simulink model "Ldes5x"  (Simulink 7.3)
settings: Solver=ode45  StartTime=0.0  StopTime=10.0  RelTol=1e-3
undefined symbols (not defined in the file or in its folder): Alv, Blv, Clv, Dlv

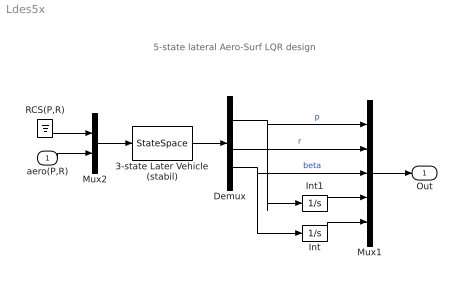
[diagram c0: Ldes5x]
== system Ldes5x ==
  note: 5-state lateral Aero-Surf LQR design
  aero(P,R) : Inport  OutDataType=sfix(16)  OutScaling=2^0
  3-state Later Vehicle (stabil) : StateSpace  A=Alv  B=Blv  C=Clv  D=Dlv
  Demux : Demux  Outputs=3
  Int : Integrator
  Int1 : Integrator
  Mux1 : Mux  Inputs=5
  Mux2 : Mux  Inputs=[2, 2]
  RCS(P,R) : Ground
  Out : Outport  OutDataType=sfix(16)  OutScaling=2^0
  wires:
  3-state Later Vehicle (stabil)/1 -> Demux/1
  Demux/1 -> Mux1/1, Int1/1  "p"
  Demux/2 -> Mux1/2  "r"
  Mux1/1 -> Out/1
  Mux2/1 -> 3-state Later Vehicle (stabil)/1
  aero(P,R)/1 -> Mux2/2
  RCS(P,R)/1 -> Mux2/1
  Demux/3 -> Int/1, Mux1/3  "beta"
  Int/1 -> Mux1/5
  Int1/1 -> Mux1/4
